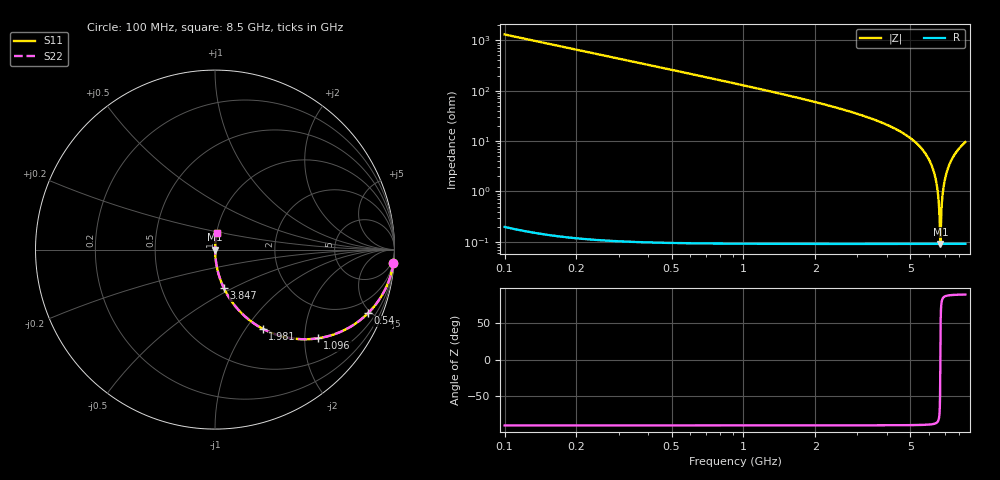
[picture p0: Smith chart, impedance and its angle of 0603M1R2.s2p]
! Created Wed Apr 18 13:44:53 2012
# hz S ma R 50
! 2 Port Network Data from SP1.SP block
! freq  magS11  angS11  magS21  angS21  magS12  angS12  magS22  angS22
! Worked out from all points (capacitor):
!   8401 points, 100 MHz to 8.5 GHz, reference 50 ohm
!   read as one part in series: C = 1.22 pF near 142 MHz
!   lowest |Z| = 91.2 mohm at 6.676 GHz (marker M1)
!   series resonance near 6.676 GHz, so ESL is about 470 pH
!   S11 on the Smith chart (normalised r, x): 100 MHz: 1, -26; 540 MHz: 1.00, -4.80; 1.096 GHz: 1.00, -2.32; 1.981 GHz: 1.00, -1.20; 3.847 GHz: 1.00, -0.45; 8.5 GHz: 1.00, +0.19
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1e8  0.9971 -4.4  0.07645 85.6  0.07645 85.6  0.9971 -4.4
2.8e8  0.9776 -12.1  0.2102 77.9  0.2102 77.9  0.9776 -12.1
5.4e8  0.923 -22.6  0.3846 67.4  0.3846 67.4  0.923 -22.6
1.096e9  0.7566 -40.8  0.6533 49.2  0.6533 49.2  0.7566 -40.8
1.5e9  0.6364 -50.4  0.7706 39.5  0.7706 39.5  0.6364 -50.4
1.981e9  0.5145 -58.9  0.8567 31.0  0.8567 31.0  0.5145 -58.9
2.9e9  0.3427 -69.8  0.9386 20.0  0.9386 20.0  0.3427 -69.8
3.847e9  0.2208 -77.0  0.9744 12.8  0.9744 12.8  0.2208 -77.0
4.3e9  0.1747 -79.6  0.9837 10.1  0.9837 10.1  0.1747 -79.6
5.7e9  0.06191 -85.6  0.9972 3.5  0.9972 3.5  0.06191 -85.6
6.127e9  0.03357 -86.5  0.9985 1.9  0.9985 1.9  0.03357 -86.5
6.405e9  0.01621 -85.9  0.999 0.9  0.999 0.9  0.01621 -85.9
6.557e9  0.007073 -82.2  0.9991 0.4  0.9991 0.4  0.007073 -82.2
6.603e9  0.004376 -77.7  0.9991 0.2  0.9991 0.2  0.004376 -77.7
6.651e9  0.001711 -57.7  0.9991 0.1  0.9991 0.1  0.001711 -57.7
6.676e9  0.0009114 1.2  0.9991 -0.0  0.9991 -0.0  0.0009114 1.2
6.702e9  0.001789 59.3  0.9991 -0.1  0.9991 -0.1  0.001789 59.3
6.766e9  0.005336 79.9  0.9991 -0.3  0.9991 -0.3  0.005336 79.9
6.83e9  0.008987 83.7  0.999 -0.5  0.999 -0.5  0.008987 83.7
7.1e9  0.02413 86.5  0.9988 -1.4  0.9988 -1.4  0.02413 86.5
7.638e9  0.05279 86.0  0.9977 -3.0  0.9977 -3.0  0.05279 86.0
8.5e9  0.09508 84.0  0.9946 -5.5  0.9946 -5.5  0.09508 84.0
